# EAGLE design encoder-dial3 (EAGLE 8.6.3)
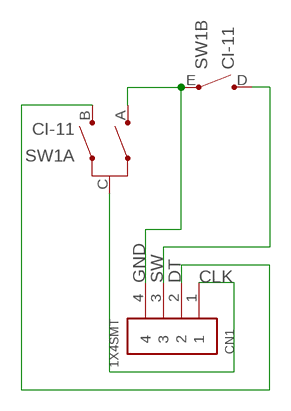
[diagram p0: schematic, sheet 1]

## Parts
CN1  1X4SMT  [1X4-SMT]
SW1  CI-11  [CI-11]

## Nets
CLK: CN1.1 SW1.C(A:C)
DT: CN1.2 SW1.B(A:B)
GND: CN1.4 SW1.A(A:A) SW1.E(B:E)
SW: CN1.3 SW1.D(B:D)

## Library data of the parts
CN1 = adafruit:1X4: 4-pin connector
SW1 = piher:CI-11: 11mm Incemental Encoder Source: www.piher.net .. 04-CI-11v04.pdf; OC_FARNELL: unknown; OC_NEWARK: unknown

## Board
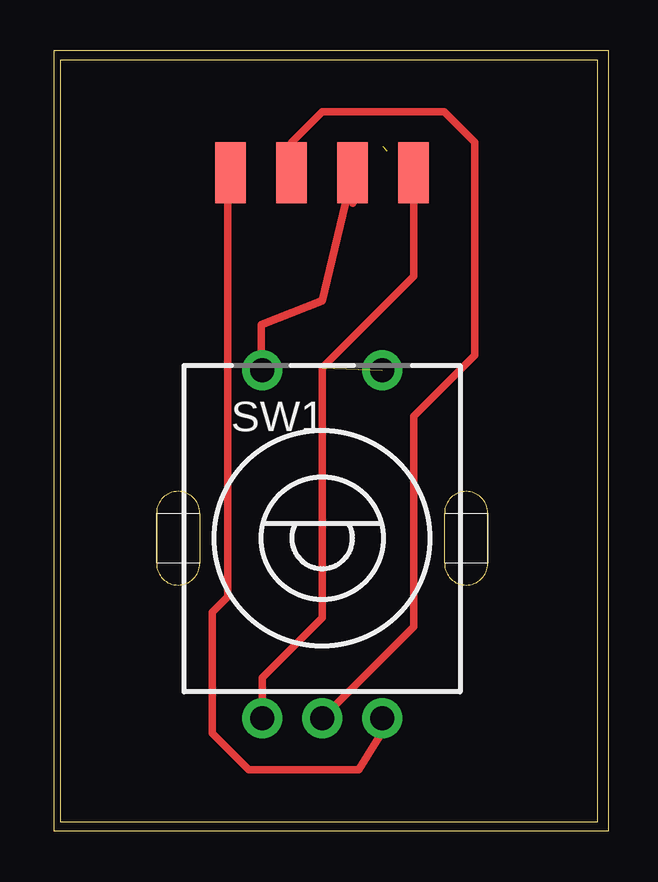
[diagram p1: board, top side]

Size 22.4 x 31.74 mm. Coordinates in mm from the lower left corner, seen from the top.
Outline: 0,0 22.4,0 22.4,31.74 0,31.74 0,0
Copper layers (1*16): Top 0.035mm / dielectric 1.5mm / Bottom 0.035mm
Design rules "default": minimum track width 6mil, minimum drill 0.35mm, track to track 6mil, track to pad 6mil, pad to pad 6mil, via to via 6mil, smd to smd 6mil, copper to edge 40mil, drill to drill 6mil, minimum pad ring 10mil, minimum via ring 8mil, stop-mask expansion 4mil, vias tented up to drill 0mil, thermal gap 10mil
Milling: area -0.3,-0.4 to 22.9,32.1

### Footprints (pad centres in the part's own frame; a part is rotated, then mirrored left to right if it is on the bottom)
1X4-SMT = smd 1.27 x 2.54: 1 -3.81,0; 2 -1.27,0; 3 1.27,0; 4 3.81,0
CI-11 = drill 1 pad 1.676: A -2.5,-7.5; B 0,-7.5; C 2.5,-7.5; D -2.5,7; E 2.5,7

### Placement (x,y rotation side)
CN1  10.92,27.05 0 top
SW1  10.92,11.81 0 top

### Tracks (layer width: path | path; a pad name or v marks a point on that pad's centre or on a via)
CLK
  Top 0.305: CN1.1 6.99,26.93 6.99,9.38 6.35,8.74 6.35,3.68 7.87,2.16 12.45,2.16 13.68,4.15 SW1.C
DT
  Top 0.305: CN1.2 9.65,28.32 10.92,29.59 16,29.59 17.27,28.32 17.27,19.43 14.73,16.89 14.73,8.12 SW1.B
GND  (1 unrouted)
  Top 0.305: CN1.4 14.73,22.73 10.92,18.92 10.92,8.51 8.42,6.01 SW1.A
N$1  (1 unrouted)
SW
  Top 0.305: 12.19,25.78 CN1.3 10.92,21.72 8.38,20.7 8.38,18.85 SW1.D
